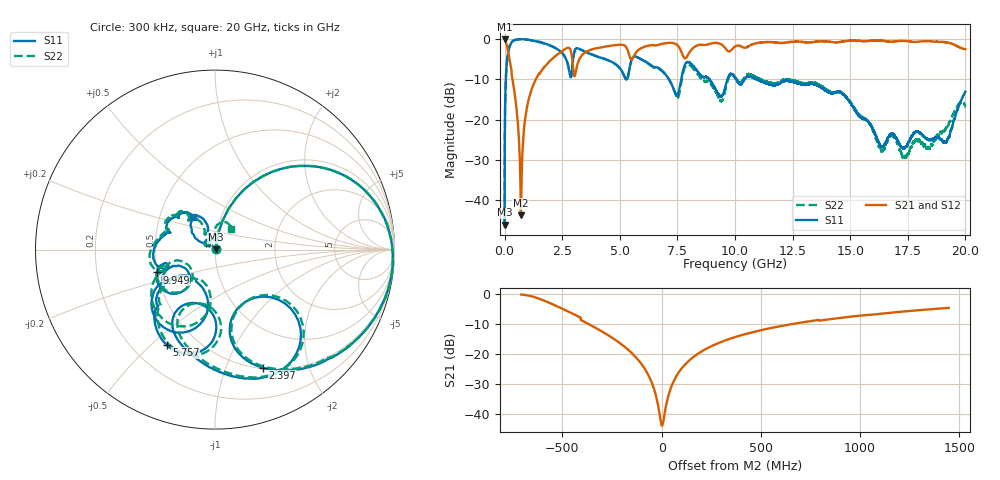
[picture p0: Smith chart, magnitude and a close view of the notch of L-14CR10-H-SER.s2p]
!{L-14CR10}
!Johanson Technology Inc.
!www.johansontechnology.com
!Test Board Conditions:
!Substrate Type  RO4350B
!Substrate Thickness  20 mil
!Substrate Dk  3.66
!TL Type: GCPW
!TL Trace Width  36 mil
!TL Gap  12 mil
!Electrode orientation  Horizontal
!DUT TOPOLOGY	SERIES
!Mounting Pad LxW  26x36 mil
! Created Sun Jun 20 13:09:14 2021
# hz S ma R 50
! 2 Port Network Data from SP1.SP block
! freq  magS11  angS11  magS21  angS21  magS12  angS12  magS22  angS22
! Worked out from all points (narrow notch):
!   20001 points, 300 kHz to 20 GHz, reference 50 ohm
!   highest |S21| = -0.02 dB at 1.3 MHz (marker M1); lowest = -43.7 dB at 707.3 MHz (marker M2)
!   notch at M2: 42.5 dB deep, 241 MHz wide at half that depth
!   lowest |S11| = -46.0 dB at 300 kHz (marker M3), VSWR 1.01, Z = 50.5 + j0.196 ohm
!   |S11| at or under -10 dB: 7.134 GHz to 7.668 GHz (533.5 MHz wide, 7.21 % of centre); 8.889 GHz to 9.671 GHz (781.3 MHz wide, 8.42 % of centre); 10.95 GHz to end of sweep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
!   |S22| runs from -46.8 to -0.1 dB; largest |S21 - S12| = 0.013
!   S11 on the Smith chart (normalised r, x): 300 kHz: 1.01, +0.00; 2.397 GHz: 0.51, -1.36; 5.757 GHz: 0.34, -0.56; 9.949 GHz: 0.50, -0.14; 20 GHz: 0.73, +0.28
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300000  0.004984 23.0  0.9959 -0.2  0.9951 -0.2  0.00459 20.4
1300000  0.00909 72.2  0.9974 -0.5  0.9968 -0.6  0.009284 71.0
1.033e8  0.5342 53.9  0.8179 -33.3  0.819 -33.3  0.5359 53.8
1.563e8  0.6935 42.2  0.6894 -45.6  0.6924 -45.4  0.6963 42.1
7.073e8  0.9933 -6.1  0.006496 -16.3  0.006593 -15.1  0.9938 -6.1
1.1753e9  0.9615 -24.6  0.2388 63.9  0.2391 63.7  0.9627 -24.7
2.3973e9  0.7107 -67.9  0.676 20.3  0.676 20.3  0.7099 -67.0
2.9013e9  0.3586 -47.4  0.6579 -24.4  0.6583 -24.4  0.3569 -45.8
3.3343e9  0.7321 -78.1  0.6179 8.1  0.6192 8.1  0.7322 -76.0
5.2153e9  0.3378 -117.0  0.8269 -47.0  0.8264 -46.9  0.334 -113.9
5.7573e9  0.5951 -117.0  0.7084 -35.4  0.7096 -35.4  0.5927 -114.0
6.6673e9  0.4391 -137.9  0.8461 -54.5  0.8472 -54.4  0.4285 -136.3
7.4973e9  0.1956 -122.0  0.8426 -80.4  0.843 -80.4  0.1963 -119.7
8.0183e9  0.5124 -128.9  0.6797 -65.8  0.6832 -65.6  0.4779 -131.8
9.3913e9  0.1934 -143.0  0.8641 -99.4  0.866 -99.4  0.1695 -147.8
9.9493e9  0.3486 -158.6  0.7844 -95.9  0.7883 -95.9  0.3497 -156.8
1.00003e10  0.331 -161.8  0.8057 -97.1  0.8071 -97.0  0.3367 -159.8
1.33343e10  0.2779 134.8  0.9114 -143.4  0.9092 -143.3  0.2901 135.3
1.66673e10  0.06125 154.1  0.928 168.3  0.9277 168.5  0.05983 155.7
1.73533e10  0.04455 145.0  0.9465 159.1  0.9463 159.1  0.03476 144.9
1.91253e10  0.05268 127.7  0.9145 131.9  0.917 131.9  0.07555 85.6
2e10  0.2223 123.9  0.7471 124.6  0.7427 124.7  0.1451 51.2
